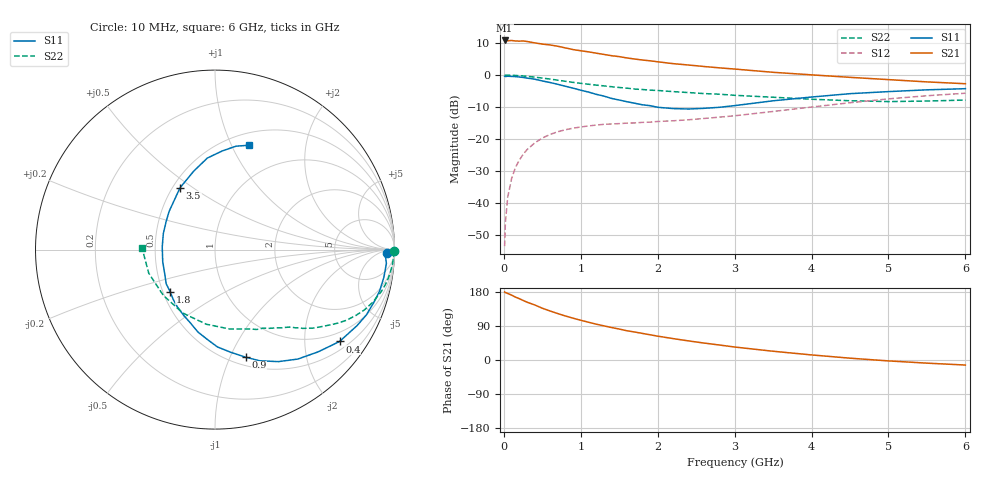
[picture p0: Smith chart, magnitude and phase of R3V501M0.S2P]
! SIEMENS Small Signal Semiconductors
! BFR181
! Si NPN RF Bipolar Junction Transistor in SOT23
! VCE = 0.5 V  IC = 1 mA
! Common Emitter S-Parameters:  May  1996
# GHz  S  MA  R  50
!  f  S11  S21  S12  S22
! GHz  MAG  ANG  MAG  ANG  MAG  ANG  MAG  ANG
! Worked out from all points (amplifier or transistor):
!   36 points, 10 MHz to 6 GHz, reference 50 ohm
!   highest |S21| = 10.8 dB at 10 MHz (marker M1)
!   |S21| within 3 dB of that: start of sweep to 940.5 MHz
!   unconditionally stable (mu >= 1): 1.805 GHz to 4.43 GHz
!   at 250 MHz: K = 0.17, MSG = 17.8 dB, |S12| = -24.9 dB
!   at 1.4 GHz: K = 0.82, MSG = 10.7 dB, |S12| = -15.3 dB
!   at 6 GHz: K = 0.97, MSG = 1.5 dB, |S12| = -5.7 dB
!   S11 on the Smith chart (normalised r, x): 10 MHz: 39, -18; 400 MHz: 0.72, -2.88; 900 MHz: 0.58, -1.15; 1.8 GHz: 0.55, -0.29; 3.5 GHz: 0.55, +0.45; 6 GHz: 0.63, +1.17
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0.01  0.959 -1.1  3.481 179.5  0.0021 87.3  0.9968 -0.5
0.02  0.95 -1.9  3.444 178.1  0.0049 85.9  0.9971 -1.0
0.05  0.958 -4.6  3.442 175.6  0.0122 86.9  0.9949 -2.5
0.1  0.9535 -9.4  3.475 171.3  0.0238 83.8  0.9919 -4.8
0.2  0.9324 -18.5  3.398 161.9  0.0464 77.6  0.9777 -9.6
0.25  0.9183 -23.4  3.419 157.2  0.0572 74.7  0.9681 -11.8
0.3  0.8974 -28.2  3.358 152.7  0.0678 72.0  0.9566 -14.0
0.4  0.8625 -36.4  3.193 145.4  0.0864 66.4  0.928 -18.3
0.5  0.8095 -44.7  3.054 136.6  0.1033 61.6  0.8984 -21.9
0.6  0.7647 -52.9  2.96 129.4  0.1176 57.4  0.8659 -25.1
0.7  0.7171 -60.5  2.827 122.6  0.1296 53.5  0.8319 -28.2
0.9  0.6241 -74.0  2.507 110.3  0.1474 47.1  0.7688 -33.0
1.1  0.5423 -88.6  2.308 99.7  0.1597 42.4  0.7188 -37.0
1.4  0.4311 -108.5  2.009 85.7  0.1717 37.8  0.6574 -41.9
1.6  0.3826 -123.1  1.852 77.2  0.1771 36.6  0.6241 -44.3
1.8  0.3426 -136.9  1.721 70.2  0.1818 36.5  0.5941 -46.7
2.2  0.299 -166.9  1.51 56.5  0.1926 37.0  0.5507 -52.4
2.8  0.3129 150.8  1.298 39.6  0.2194 39.4  0.5022 -62.4
3.5  0.3957 119.5  1.105 23.1  0.2695 40.7  0.45 -79.5
4.5  0.5117 94.8  0.921 4.8  0.3688 35.8  0.3963 -116.9
5.5  0.5875 78.6  0.782 -8.3  0.4748 24.4  0.3918 -160.4
6  0.6123 71.8  0.732 -13.3  0.5199 17.3  0.4065 178.8
